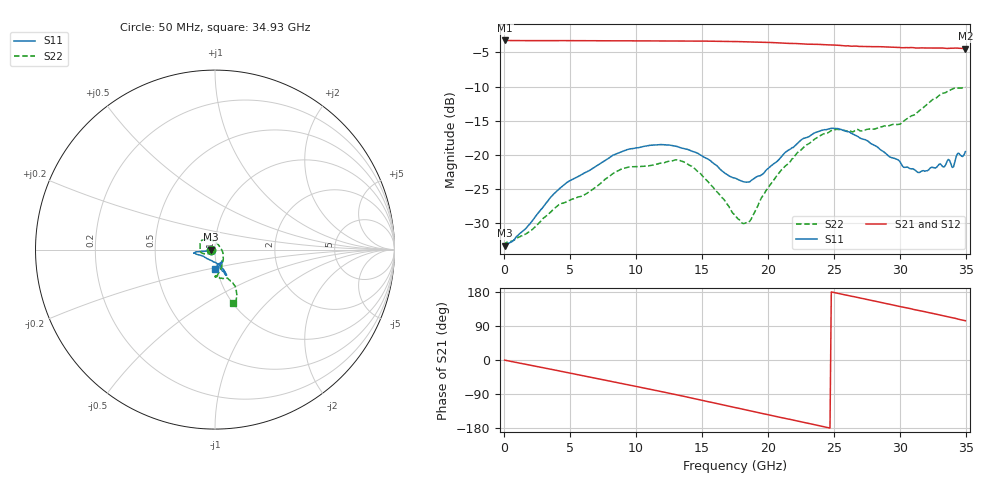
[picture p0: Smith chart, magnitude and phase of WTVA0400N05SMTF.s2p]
! 50 ohm 2-Port S-parameters measured by Modelithics Inc support@modelithics.com  Tampa, FL USA 813-866-6335 (February 2024)
! Smiths Interconnect,  4dB P/N: WTVA0400N05SMTF, Temperature: 75 C
! Board: 10 mil Rogers 4350B, Mounting Pad Dimensions: Length: 15 mils, Width: 25 mils, Gap: 40 mils.
# Hz S RI R 50
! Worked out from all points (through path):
!   352 points, 50 MHz to 34.93 GHz, reference 50 ohm
!   highest |S21| = -3.24 dB at 100 MHz (marker M1); lowest = -4.5 dB at 34.93 GHz (marker M2)
!   group delay of S21, straight-line fit = 20.5 ps
!   lowest |S11| = -33.3 dB at 50 MHz (marker M3), VSWR 1.04, Z = 47.9 + j0.052 ohm
!   |S11| at or under -10 dB: start of sweep to end of sweep
!   |S22| runs from -33.4 to -10.1 dB; largest |S21 - S12| = 0.0079
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5e7  -0.0216 0.000542  0.6885 -0.00374  0.6875 -0.00362  -0.0215 -0.00101
1e8  -0.0222 -0.000252  0.6885 -0.00853  0.6876 -0.00859  -0.0225 -0.000948
2.0905e9  -0.0323 -0.00345  0.6648 -0.1705  0.6639 -0.1706  -0.0271 -0.00772
4.2795e9  -0.0568 -0.00948  0.5977 -0.3382  0.5966 -0.3379  -0.0388 -0.0203
5.8715e9  -0.0711 -0.00979  0.5209 -0.4469  0.5202 -0.4466  -0.044 -0.0235
8.8565e9  -0.1044 -0.0123  0.3257 -0.6017  0.3238 -0.6016  -0.0767 -0.0173
1.1742e10  -0.1174 -0.0194  0.0926 -0.6761  0.091 -0.6755  -0.0837 0.0224
1.30355e10  -0.114 -0.0198  -0.0193 -0.682  -0.0206 -0.6813  -0.0804 0.0451
1.42295e10  -0.1037 -0.0249  -0.1249 -0.6706  -0.1264 -0.6696  -0.061 0.0556
1.7513e10  -0.0462 -0.0494  -0.39 -0.5523  -0.3901 -0.5511  0.0118 0.0339
1.811e10  -0.0318 -0.0552  -0.4314 -0.5161  -0.4308 -0.5155  0.0231 0.0214
1.86075e10  -0.0185 -0.0609  -0.4626 -0.4859  -0.463 -0.4845  0.0319 0.00726
2.0697e10  0.0252 -0.0866  -0.5719 -0.3339  -0.5716 -0.3329  0.0459 -0.0547
2.33835e10  0.0599 -0.1295  -0.6365 -0.115  -0.6358 -0.1148  0.0214 -0.1259
2.5473e10  0.0596 -0.1422  -0.63 0.0646  -0.6291 0.0648  0.00226 -0.1533
2.91545e10  0.0291 -0.0929  -0.5192 0.3323  -0.5152 0.3369  0.0388 -0.1591
3.1443e10  0.0374 -0.0643  -0.3951 0.4604  -0.3921 0.4617  0.1002 -0.1857
3.33335e10  0.029 -0.0766  -0.2642 0.5438  -0.2608 0.5446  0.1176 -0.2586
3.3632e10  0.032 -0.087  -0.2445 0.5509  -0.2395 0.5524  0.1197 -0.2694
3.39305e10  0.0253 -0.077  -0.2233 0.5612  -0.2187 0.5621  0.1182 -0.2795
3.43285e10  0.0164 -0.101  -0.1893 0.5741  -0.1858 0.5744  0.1063 -0.2898
3.49255e10  -0.00102 -0.1057  -0.1418 0.5819  -0.1411 0.5809  0.0981 -0.2985
